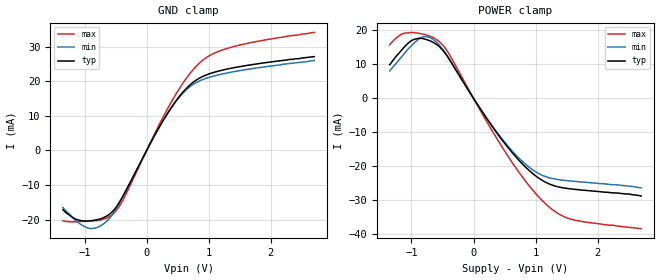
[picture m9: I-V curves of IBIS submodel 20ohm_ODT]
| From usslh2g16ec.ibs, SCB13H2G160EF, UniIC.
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| SUBMODEL 20ohm_ODT
[Submodel]   20ohm_ODT
Submodel_type  Dynamic_clamp
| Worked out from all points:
|   GND clamp passes 1 mA (typ) near -0.03 V on its own axis
[GND Clamp]
|Voltage   I(typ)   I(min)   I(max)
-1.35V    -17.1mA    -16.5mA    -20.3mA
-1.15V    -19.8mA    -20.2mA    -20.6mA
-950mV    -20.4mA    -22.4mA    -20.4mA
-650mV    -19.03mA   -20.58mA   -19.57mA
-500mV    -16.62mA   -17.18mA   -17.61mA
-400mV    -13.77mA   -13.96mA   -14.92mA
100mV     3.414mA    3.411mA    3.769mA
400mV     12.47mA    12.37mA    14.07mA
650mV     18.12mA    17.72mA    21.11mA
900mV     21.34mA    20.45mA    26.02mA
1.45V     24.05mA    22.9mA     30.23mA
2.7V      27.1mA     26mA       34.1mA
[POWER Clamp]
|Voltage   I(typ)   I(min)   I(max)
-1.35V    9.9mA      8.1mA      15.8mA
-1.15V    14.4mA     12.4mA     19mA
-1V       17mA       15.5mA     19.4mA
-850mV    17.7mA     17.8mA     19mA
-700mV    16.92mA    17.86mA    18.28mA
-550mV    15.2mA     15.66mA    16.66mA
-400mV    11.77mA    11.79mA    13.23mA
500mV     -13.18mA   -12.83mA   -15.45mA
850mV     -20.42mA   -19.55mA   -24.63mA
1.15V     -24.56mA   -22.93mA   -30.83mA
1.6V      -26.68mA   -24.35mA   -35.66mA
2.7V      -28.7mA    -26.3mA    -38.3mA
